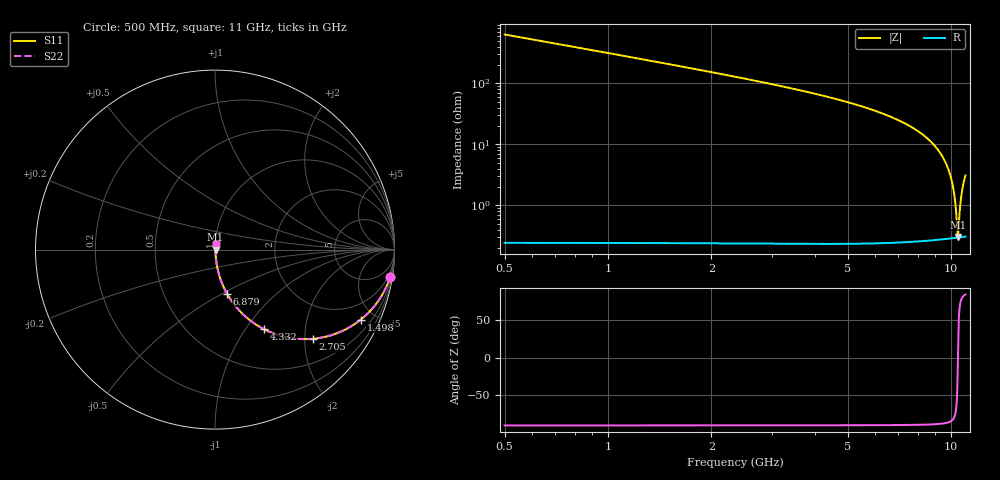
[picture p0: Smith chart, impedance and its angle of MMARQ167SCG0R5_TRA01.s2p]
! MMARQ167SCG0R5_TRA01  S-PARAMETER MODEL  ( General Type )
! Model Generated by TAIYO YUDEN Corporation (http://www.ty-top.com)
! Version 1.0
! TAIYO YUDEN Control No. 160201
! Copyright(c) 2016 TAIYO YUDEN CO.,LTD. All Rights Reserved.
! Product Description (link to TY-COMPAS)
! https://ds.yuden.co.jp/TYCOMPAS/or/detail?pn=MMARQ167SCG0R5BTRA01&u=M
! Products Name : Multilayer Ceramic Capacitors
! Characteristics :
!  Capacitance : 0.5 pF , Rated Voltage : 250V , TCC : CG / C0G
!  Case Size : 1.6 x 0.8 / 0.063 x 0.031 [mm/inch] , Thickness : 0.7 / 0.028 [mm/inch]
!  (Conditions: Temperature = 25 degC , DC Bias Current/Voltage = 0A / 0V)
! External Node Assignments :
!  1  o---| |---o  2
! GND o---------o GND
! Frequency Range : 500MHz  -  11000MHz  [ 401 STEP ]
# MHz S RI R 50
! Freq[MHz].  S11 Real  S11 Imag  S21 Real  S21 Imag  S12 Real  S12 Imag  S22 Real  S22 Imag
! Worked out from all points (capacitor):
!   401 points, 500 MHz to 11 GHz, reference 50 ohm
!   read as one part in series: C = 499 fF near 552.5 MHz
!   lowest |Z| = 304 mohm at 10.45 GHz (marker M1)
!   series resonance near 10.46 GHz, so ESL is about 460 pH
!   S11 on the Smith chart (normalised r, x): 500 MHz: 1, -13; 1.498 GHz: 1.00, -4.17; 2.705 GHz: 1.00, -2.20; 4.332 GHz: 1.00, -1.22; 6.879 GHz: 1.00, -0.53; 11 GHz: 1.01, +0.06
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500  0.9758 -0.1534  0.0242 0.1534  0.0242 0.1534  0.9758 -0.1534
946.25  0.9176 -0.2746  0.0824 0.2746  0.0824 0.2746  0.9176 -0.2746
1497.5  0.8126 -0.3896  0.1874 0.3896  0.1874 0.3896  0.8126 -0.3896
2258.75  0.6439 -0.478  0.3561 0.478  0.3561 0.478  0.6439 -0.478
2705  0.5472 -0.4967  0.4528 0.4967  0.4528 0.4967  0.5472 -0.4967
4017.5  0.3145 -0.4626  0.6855 0.4626  0.6855 0.4626  0.3145 -0.4626
4332.5  0.2717 -0.4429  0.7283 0.4429  0.7283 0.4429  0.2717 -0.4429
5750  0.1318 -0.3352  0.8682 0.3352  0.8682 0.3352  0.1318 -0.3352
6878.75  0.0667 -0.2449  0.9333 0.2449  0.9333 0.2449  0.0667 -0.2449
7508.75  0.0429 -0.1965  0.9571 0.1965  0.9571 0.1965  0.0429 -0.1965
8532.5  0.0179 -0.1225  0.9821 0.1225  0.9821 0.1225  0.0179 -0.1225
9267.5  0.00814 -0.0732  0.9919 0.0732  0.9919 0.0732  0.00814 -0.0732
9740  0.0047 -0.0432  0.9953 0.0432  0.9953 0.0432  0.0047 -0.0432
10055  0.00346 -0.0239  0.9965 0.0239  0.9965 0.0239  0.00346 -0.0239
10265  0.00305 -0.0114  0.9969 0.0114  0.9969 0.0114  0.00305 -0.0114
10422.5  0.00296 -0.00218  0.997 0.00218  0.997 0.00218  0.00296 -0.00218
10448.75  0.00296 -0.00065  0.997 0.00065  0.997 0.00065  0.00296 -0.00065
10501.25  0.00297 0.00239  0.997 -0.00239  0.997 -0.00239  0.00297 0.00239
10606.25  0.00306 0.00842  0.9969 -0.00842  0.9969 -0.00842  0.00306 0.00842
10711.25  0.00322 0.0144  0.9968 -0.0144  0.9968 -0.0144  0.00322 0.0144
10842.5  0.00351 0.0218  0.9965 -0.0218  0.9965 -0.0218  0.00351 0.0218
11000  0.004 0.0305  0.996 -0.0305  0.996 -0.0305  0.004 0.0305
